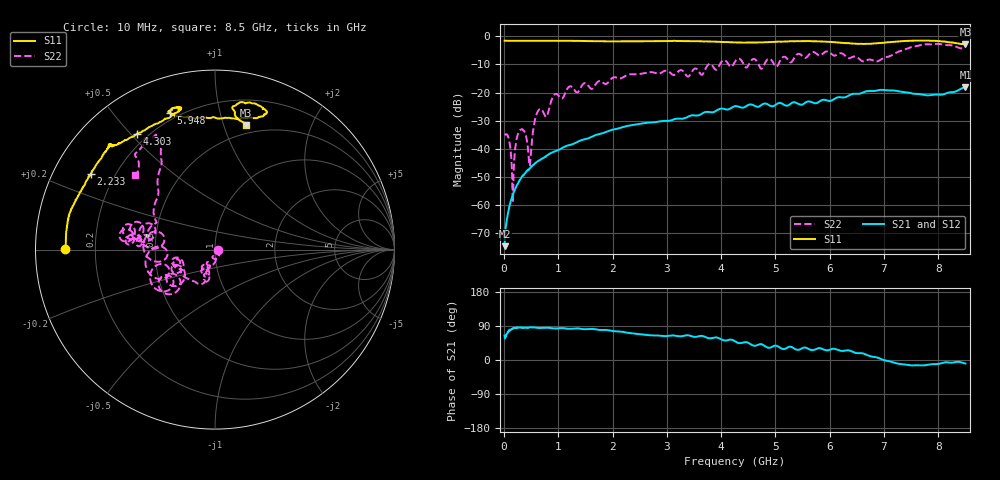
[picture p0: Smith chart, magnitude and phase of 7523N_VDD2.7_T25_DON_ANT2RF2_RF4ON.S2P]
!Agilent Technologies,E5071C,MY46417908,A.11.23
!Date: Wed Dec 09 17:50:16 2020
!Data & Calibration Information:
!Freq	S11:SOLT2(ON)	S21:SOLT2(ON)	S12:SOLT2(ON)	S22:SOLT2(ON)
!PortZ  Port1:50+j0  Port2:50+j0
!Above PortZ is port z conversion or system Z0 setting when saving the data.
!When reading, reference impedance value at option line is always used.
# Hz S dB R 50
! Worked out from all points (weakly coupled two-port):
!   1601 points, 10 MHz to 8.5 GHz, reference 50 ohm
!   highest |S21| = -18.10 dB at 8.5 GHz (marker M1); lowest = -74.5 dB at 10 MHz (marker M2)
!   lowest |S11| = -2.9 dB at 8.5 GHz (marker M3), VSWR 6.03, Z = 21 + j59.7 ohm
!   |S11| at or under -10 dB: nowhere
!   |S22| runs from -59.0 to -2.7 dB; largest |S21 - S12| = 0.0011
!   S11 on the Smith chart (normalised r, x): 10 MHz: 0.09, +0.00; 2.233 GHz: 0.11, +0.28; 4.303 GHz: 0.16, +0.52; 5.948 GHz: 0.17, +0.71; 8.5 GHz: 0.42, +1.19
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1e7  -1.57 179.7  -74.53 64.6  -73.09 60.0  -35.10 -3.8
7.898125e7  -1.59 178.5  -62.27 73.6  -62.20 74.5  -35.83 -39.3
1.638812e8  -1.59 176.9  -56.36 82.6  -56.20 82.9  -58.98 31.4
2.381688e8  -1.58 175.7  -52.82 84.8  -52.85 85.8  -35.90 37.5
2.912312e8  -1.58 174.8  -50.89 85.9  -51.03 85.8  -33.32 -1.4
3.761312e8  -1.57 173.3  -48.84 85.1  -48.83 85.6  -33.88 -64.6
4.716438e8  -1.57 171.7  -46.93 86.3  -46.95 86.2  -46.08 -61.7
6.361375e8  -1.55 169.6  -44.16 84.7  -44.20 84.9  -26.18 -79.1
7.794062e8  -1.56 168.2  -42.50 85.3  -42.49 85.6  -28.54 -99.1
9.332875e8  -1.56 166.7  -40.88 83.4  -40.88 83.4  -20.60 -107.3
1.426769e9  -1.65 162.1  -36.84 82.0  -36.87 82.0  -17.71 -110.6
2.233319e9  -1.83 148.7  -31.97 72.9  -31.96 73.0  -14.05 -108.9
2.843538e9  -1.73 137.4  -30.30 64.4  -30.28 64.5  -13.26 -150.8
4.255e9  -2.20 125.4  -24.79 49.3  -24.77 49.3  -8.98 -139.5
4.302756e9  -2.18 123.9  -24.88 45.7  -24.86 45.6  -8.01 -147.1
4.743175e9  -2.17 110.3  -24.35 41.8  -24.34 41.8  -11.52 -175.2
5.671769e9  -1.76 107.6  -23.43 26.1  -23.41 26.4  -5.63 169.2
5.947694e9  -1.92 108.1  -22.76 25.3  -22.77 25.5  -5.37 171.2
6.664038e9  -2.67 86.0  -19.56 14.6  -19.58 14.6  -8.67 171.1
7.088538e9  -2.11 70.9  -19.20 -3.0  -19.25 -3.2  -7.18 136.4
7.757125e9  -1.50 76.3  -20.89 -13.9  -20.89 -13.8  -2.87 117.2
8.5e9  -2.91 75.9  -18.10 -9.5  -18.12 -9.0  -4.33 137.1
